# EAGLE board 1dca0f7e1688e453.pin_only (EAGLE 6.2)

Size 56 x 85 mm. Coordinates in mm from the lower left corner, seen from the top.
Outline: 56,0 0,0 0,85 56,85
Copper layers (1*16): Top 0.035mm / dielectric 1.5mm / Bottom 0.035mm
Design rules: minimum track width 8mil, minimum drill 15mil, track to track 8mil, track to pad 8mil, pad to pad 8mil, via to via 8mil, smd to smd 8mil, copper to edge 1mil, drill to drill 8mil, minimum pad ring 10mil, minimum via ring 8mil, stop-mask expansion 4mil, vias tented up to drill 20mil, thermal gap 10mil

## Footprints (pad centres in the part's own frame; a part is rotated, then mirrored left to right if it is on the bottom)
1X04-3.5MM = drill 1 pad 2.184: 1 -5.25,0; 2 -1.75,0; 3 1.75,0; 4 5.25,0
1X04-CLEANBIG = drill 1.016 pad 1.778: 1 -3.81,0; 2 -1.27,0; 3 1.27,0; 4 3.81,0
1X2-3.5MM = drill 1 pad 2.184: 1 1.8,0; 2 -1.7,0
1X05-3.5MM = drill 1 pad 2.184: 1 7,0; 2 3.5,0; 3 0,0; 4 -3.5,0; 5 -7,0
1X08-3.5MM = drill 1 pad 2.184: 1 -12.25,0; 2 -8.75,0; 3 -5.25,0; 4 -1.75,0; 5 1.75,0; 6 5.25,0; 7 8.75,0; 8 12.25,0
1X08-BIG = drill 1.016 pad 1.778 octagon: 1 -8.89,0; 2 -6.35,0; 3 -3.81,0; 4 -1.27,0; 5 1.27,0; 6 3.81,0; 7 6.35,0; 8 8.89,0
1X06-BIG = drill 1.016 pad 1.778 octagon: 1 -6.35,0; 2 -3.81,0; 3 -1.27,0; 4 1.27,0; 5 3.81,0; 6 6.35,0
RASBERRYPI_SHIELD = drill 1 pad 1.676 square: 1 51.308,82.55 | drill 1 pad 1.676: 2 53.848,82.55; 3 51.308,80.01; 4 53.848,80.01; 5 51.308,77.47; 6 53.848,77.47; 7 51.308,74.93; 8 53.848,74.93; 9 51.308,72.39; 10 53.848,72.39; 11 51.308,69.85; 12 53.848,69.85; 13 51.308,67.31; 14 53.848,67.31; 15 51.308,64.77; 16 53.848,64.77; 17 51.308,62.23; 18 53.848,62.23; 19 51.308,59.69; 20 53.848,59.69; 21 51.308,57.15; 22 53.848,57.15; 23 51.308,54.61; 24 53.848,54.61; 25 51.308,52.07; 26 53.848,52.07
SO-16NMW = smd 0.635 x 4.445: P$1 -3.048,-3.683; P$2 -1.778,-3.683; P$3 -0.508,-3.683; P$4 0.762,-3.683; P$5 2.032,-3.683; P$6 3.302,-3.683; P$7 4.572,-3.683; P$8 5.842,-3.683; P$9 5.842,3.429; P$10 4.572,3.429; P$11 3.302,3.429; P$12 2.032,3.429; P$13 0.762,3.429; P$14 -0.508,3.429; P$15 -1.778,3.429; P$16 -3.048,3.429

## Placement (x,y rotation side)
CN1  1X4-3.5MM  [1X04-3.5MM]  36.79,79.47 180 top
CN2  1X4-3.5MM  [1X04-3.5MM]  5.79,27 270 top
CN3  1X4-3.5MM  [1X04-3.5MM]  47.5,3.81 0 top
CN4  1X4-CLEANBIG  [1X04-CLEANBIG]  46.74,9.4 180 top
J1  1X2-3.5MM  [1X2-3.5MM]  5.79,78 270 top
J2  1X2-3.5MM  [1X2-3.5MM]  5.79,69.5 270 top
J3  1X5  [1X05-3.5MM]  19.29,79.47 180 top
JP1  [1X08-3.5MM]  5.79,50 270 top
JP2  [1X08-BIG]  11.18,45.72 90 top
JP3  [1X06-BIG]  11.18,66.04 270 top
JP4  [1X08-BIG]  29.46,74.17 180 top
JP5  [1X08-BIG]  1.27,10.16 90 top
JP6  [1X08-BIG]  17.78,10.16 270 top
U$1  RASPBERRYPI_BB  [RASBERRYPI_SHIELD]  0,0 0 top
U$2  SMD-16SOIC  [SO-16NMW]  9.4,8.64 90 top
U$3  [ADAFRUIT_TEXT_20MM]  19.56,2.79 0 top

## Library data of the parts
CN1-CN4 J1-J3 JP1-JP6 = adafruit
U$1 U$3 = microbuilder
U$2 = boogie

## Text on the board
Bottom: Copyright (c) 2012 | Adafruit Industries | Licenced under | CERN OHL v1.1 | http://ohwr.org/cernohl
tPlace: CS1 | CS0 | SCLK | MISO | MOSI | 5V | GND | GND | 3.3V | SDA | SCL | TXD | CS1 | CS0 | CLK | MISO | MOSI | 5.0V | GND | 3.3V | SDA | RXD | SCL | TXD | #17 | RXD | 3.3V | #18 | GND | #21 | #22 | IO17 | IO18 | #23 | IO21 | #24 | IO22 | IO23 | #25 | IO24 | #4 | IO25 | IO4 | 5V | GND | 3V3 | GND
